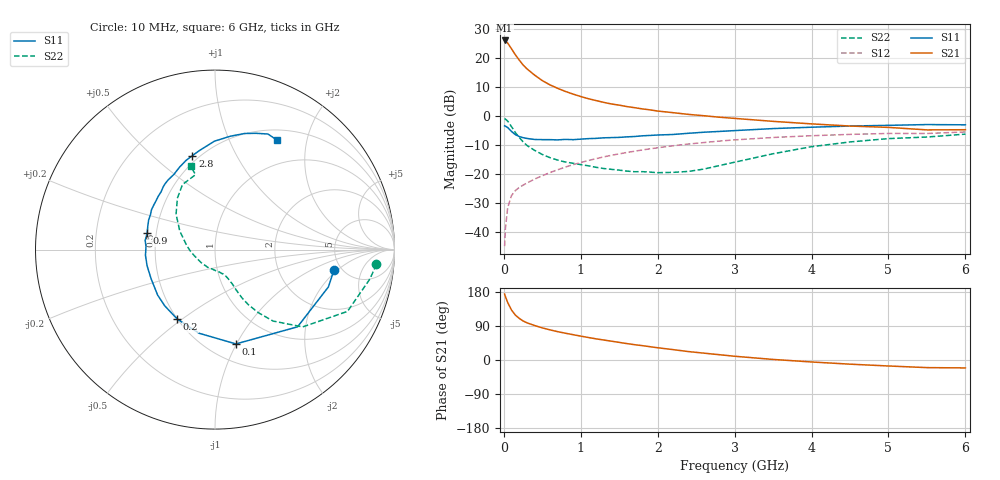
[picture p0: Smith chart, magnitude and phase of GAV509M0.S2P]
! Infineon Technologies  Discrete & RF Semiconductors
! BF775
! Si NPN RF Bipolar Junction Transistor in SOT23
! VCE = 0.5 V  IC = 9 mA
! Common Emitter S-Parameters:  May  1996
# GHz  S  MA  R  50
!  f  S11  S21  S12  S22
! GHz  MAG  ANG  MAG  ANG  MAG  ANG  MAG  ANG
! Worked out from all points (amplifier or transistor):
!   36 points, 10 MHz to 6 GHz, reference 50 ohm
!   highest |S21| = 26.1 dB at 10 MHz (marker M1)
!   |S21| within 3 dB of that: start of sweep to 102.7 MHz
!   unconditionally stable (mu >= 1): 345.2 MHz to end of sweep
!   at 250 MHz: K = 0.84, MSG = 20.8 dB, |S12| = -23.9 dB
!   at 1.4 GHz: K = 1.34, MAG = 5.4 dB, |S12| = -13.6 dB
!   at 6 GHz: K = 1.12, MAG = -1.7 dB, |S12| = -5.5 dB
!   S11 on the Smith chart (normalised r, x): 10 MHz: 4.37, -1.78; 100 MHz: 0.67, -0.99; 200 MHz: 0.50, -0.48; 900 MHz: 0.45, +0.10; 2.8 GHz: 0.46, +0.68; 6 GHz: 0.63, +1.52
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0.01  0.6733 -9.5  20.15 174.0  0.0056 82.0  0.9035 -5.2
0.02  0.6652 -18.2  19.83 167.6  0.0112 78.9  0.8787 -10.7
0.05  0.6298 -43.1  18.16 151.8  0.026 69.4  0.8145 -25.0
0.1  0.5383 -77.5  14.45 131.7  0.0421 58.1  0.6514 -41.4
0.15  0.4743 -100.9  11.37 118.5  0.0512 52.0  0.513 -50.9
0.2  0.4402 -118.6  9.241 109.8  0.058 50.3  0.4253 -55.6
0.25  0.4202 -131.8  7.606 103.0  0.0635 50.0  0.3563 -58.9
0.3  0.4079 -141.6  6.516 98.2  0.0691 51.2  0.3087 -60.8
0.4  0.3912 -155.7  5.072 91.0  0.081 52.9  0.2538 -62.3
0.5  0.3889 -166.6  4.078 84.8  0.0924 54.5  0.2155 -63.2
0.6  0.3887 -175.2  3.436 79.5  0.1049 55.5  0.1896 -64.7
0.7  0.3849 177.4  2.996 74.8  0.1172 56.2  0.1723 -66.2
0.9  0.3886 166.5  2.383 66.8  0.1436 56.2  0.1517 -68.9
1.1  0.4048 156.0  1.982 59.3  0.1695 55.2  0.1371 -74.7
1.3  0.4179 147.8  1.711 52.7  0.196 53.6  0.1231 -81.6
1.6  0.4342 136.6  1.449 43.3  0.2332 50.3  0.111 -95.9
2.2  0.4774 118.7  1.137 27.4  0.3045 42.4  0.1057 -133.9
2.8  0.5387 103.5  0.95 14.0  0.3668 33.7  0.1383 -176.9
3.5  0.604 90.3  0.805 1.5  0.4236 23.2  0.2218 152.2
4.5  0.6677 75.7  0.668 -11.0  0.4792 9.5  0.3547 126.2
5.5  0.7083 65.4  0.573 -20.1  0.4968 -3.3  0.4313 104.6
6  0.7014 60.6  0.577 -20.9  0.528 -6.9  0.4842 106.2
